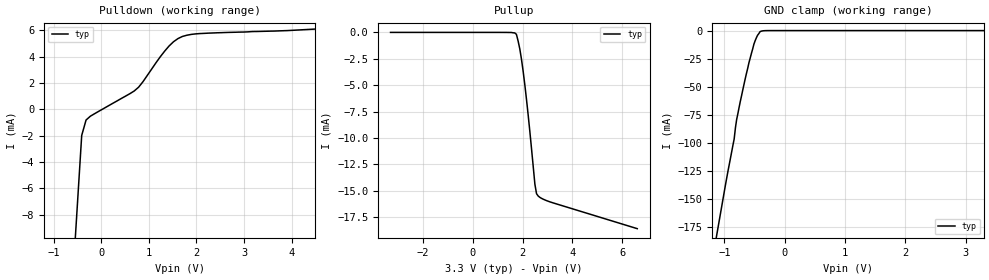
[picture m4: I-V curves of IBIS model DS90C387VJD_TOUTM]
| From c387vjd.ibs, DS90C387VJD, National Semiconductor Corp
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|   Driver Output(-)  MODEL
[Model]   DS90C387VJD_TOUTM
Model_type   3-state
| Signals   TxOUTA0- ~ TxOUTA7-; TxCLKOUT1-; TxCLKOUT2-
Vmeas = 1.2V   |This is 0.0v differential on ouput
Cref = 5pF   |Timing specification test load capacitance value
Rref = 50
Vref = 1.2
| variable   typ   min   max
C_comp   5.074pF   NA   NA
|   typ   min   max
[Temperature Range]   25.0   NA   NA
[Voltage range]   3.3V   3.0V   3.6V
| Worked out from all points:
|   slope of the pulldown table from 0 to 0.495 V, typ, clamps not added: 489 ohm
|   GND clamp passes 1 mA (typ) near -0.41 V on its own axis
[Pulldown]
| Voltage   I(typ)   I(min)   I(max)
-3.3V     -169.3mA   NA         NA
-499.6mV  -7.251mA   NA         NA
-408.6mV  -1.987mA   NA         NA
-317.2mV  -816.7uA   NA         NA
-225.7mV  -523.9uA   NA         NA
786.3mV   1.673mA    NA         NA
1.428V    4.807mA    NA         NA
1.704V    5.521mA    NA         NA
1.98V     5.716mA    NA         NA
2.439V    5.802mA    NA         NA
4.5V      6.085mA    NA         NA
6.6V      6.199mA    NA         NA
[Pullup]
| Note that the[Pullup]voltage table is referenced to Vcc
| and is calculated using Vtable=Vcc - Vmeasured.
|Voltage   I(typ)   I(min)   I(max)
-3.3V     0A         NA         NA
1.684V    -48.2uA    NA         NA
1.751V    -184.9uA   NA         NA
1.819V    -808.9uA   NA         NA
1.886V    -1.554mA   NA         NA
2.02V     -3.66mA    NA         NA
2.223V    -7.817mA   NA         NA
2.493V    -14.39mA   NA         NA
2.558V    -15.28mA   NA         NA
2.694V    -15.63mA   NA         NA
3.098V    -16.06mA   NA         NA
6.6V      -18.59mA   NA         NA
[GND_clamp]
| Outputs in Tri-state.
| Voltage   I(typ)   I(min)   I(max)
-3.3V     -852.7mA   NA         NA
-1.001V   -143.3mA   NA         NA
-838.4mV  -96.78mA   NA         NA
-816.8mV  -86.45mA   NA         NA
-797.1mV  -79.34mA   NA         NA
-654.5mV  -42.85mA   NA         NA
-593.5mV  -28.73mA   NA         NA
-511.4mV  -12.19mA   NA         NA
-450.9mV  -4.248mA   NA         NA
-408.6mV  -945.1uA   NA         NA
-265.5mV  -6.81uA    NA         NA
3.3V      0A         NA         NA
[POWER_clamp]
| Note that the[POWER_clamp]voltage table is referenced to Vcc
| and is calculated using Vtable=Vcc - Vmeasured.
| Outputs in Tri-state.
|Voltage   I(typ)   I(min)   I(max)
-3V       0A         NA         NA
3V        0A         NA         NA
[Ramp]
| Note: Ramp rate measured on single-ended Driver Output.
|   typ   min   max
dV/dt_r   180.0m/0.150n   NA   NA
dV/dt_f   181.0m/0.163n   NA   NA
R_load = 100Ohm | Note: This 100 Ohm is across the two driver output
